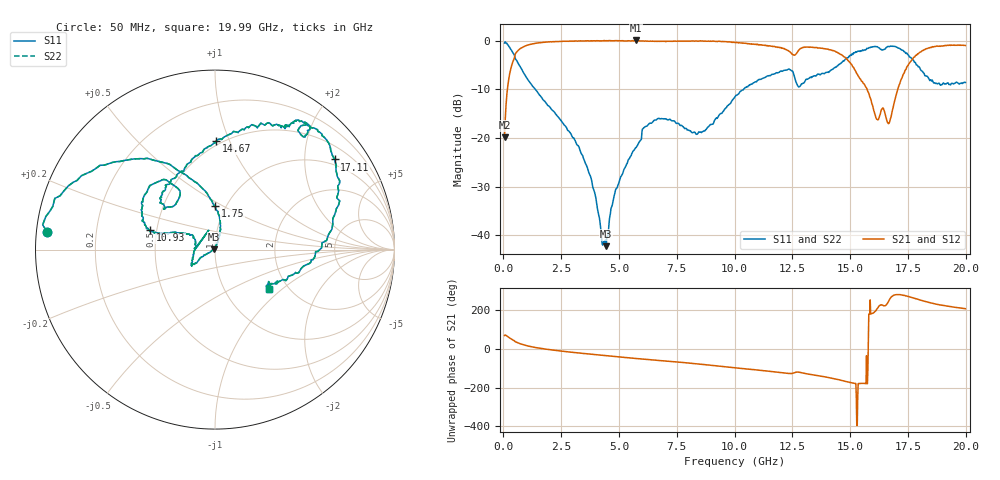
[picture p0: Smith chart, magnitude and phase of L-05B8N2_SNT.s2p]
! Data Taken on a HP 8720C VNA using a shunt-through fixture with TRL* de-embedding
#	mhz	s	ma	r	50
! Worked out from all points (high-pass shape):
!   998 points, 50 MHz to 19.99 GHz, reference 50 ohm
!   highest |S21| = 0.02 dB at 5.75 GHz (marker M1); lowest = -19.8 dB at 50 MHz (marker M2)
!   |S21| within 3 dB of the highest: 499.4 MHz to 12.55 GHz (12.05 GHz wide, 185 % of centre); 17.88 GHz to end of sweep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
!   lowest |S11| = -42.2 dB at 4.45 GHz (marker M3), VSWR 1.02, Z = 49.3 + j0.251 ohm
!   |S11| at or under -10 dB: 1.378 GHz to 10.39 GHz (9.014 GHz wide, 153 % of centre)
!   |S22| runs from -42.2 to -0.3 dB; largest |S21 - S12| = 0
!   S11 on the Smith chart (normalised r, x): 50 MHz: 0.03, +0.05; 1.75 GHz: 0.89, +0.46; 10.93 GHz: 0.46, +0.12; 14.67 GHz: 0.47, +0.89; 17.11 GHz: 0.83, +2.76; 19.99 GHz: 1.60, -0.81
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50  0.9412 173.9  0.1018 68.7  0.1018 68.7  0.9412 173.9
230  0.8741 154.6  0.4011 58.8  0.4011 58.8  0.8741 154.6
530  0.6424 128.0  0.7406 35.5  0.7406 35.5  0.6424 128.0
1750  0.2425 90.2  0.9613 -0.3  0.9613 -0.3  0.2425 90.2
3390  0.06761 70.8  0.9898 -23.3  0.9898 -23.3  0.06761 70.8
4450  0.00773 160.7  0.9954 -35.8  0.9954 -35.8  0.00773 160.7
4850  0.02913 -152.6  0.9971 -40.3  0.9971 -40.3  0.02913 -152.6
5750  0.08037 -150.5  1.002 -50.3  1.002 -50.3  0.08037 -150.5
6710  0.1584 -145.4  0.9811 -60.2  0.9811 -60.2  0.1584 -145.4
8410  0.1107 166.8  0.9872 -78.4  0.9872 -78.4  0.1107 166.8
10030  0.2654 159.0  0.9561 -98.2  0.9561 -98.2  0.2654 159.0
10930  0.3777 163.3  0.9098 -109.2  0.9098 -109.2  0.3777 163.3
13350  0.4249 134.9  0.8535 -133.9  0.8535 -133.9  0.4249 134.9
14670  0.6044 89.4  0.7016 -164.3  0.7016 -164.3  0.6044 89.4
15170  0.7471 68.6  0.5163 -178.4  0.5163 -178.4  0.7471 68.6
15350  0.7777 62.7  0.4327 -179.9  0.4327 -179.9  0.7777 62.7
15430  0.7719 61.5  0.4036 -178.9  0.4036 -178.9  0.7719 61.5
15790  0.8345 58.5  0.294 35.5  0.294 35.5  0.8345 58.5
16670  0.8689 52.8  0.1403 -113.9  0.1403 -113.9  0.8689 52.8
17110  0.8345 37.0  0.3427 -80.4  0.3427 -80.4  0.8345 37.0
18210  0.4542 -18.1  0.807 -114.2  0.807 -114.2  0.4542 -18.1
19990  0.3711 -36.2  0.8893 -153.0  0.8893 -153.0  0.3711 -36.2
